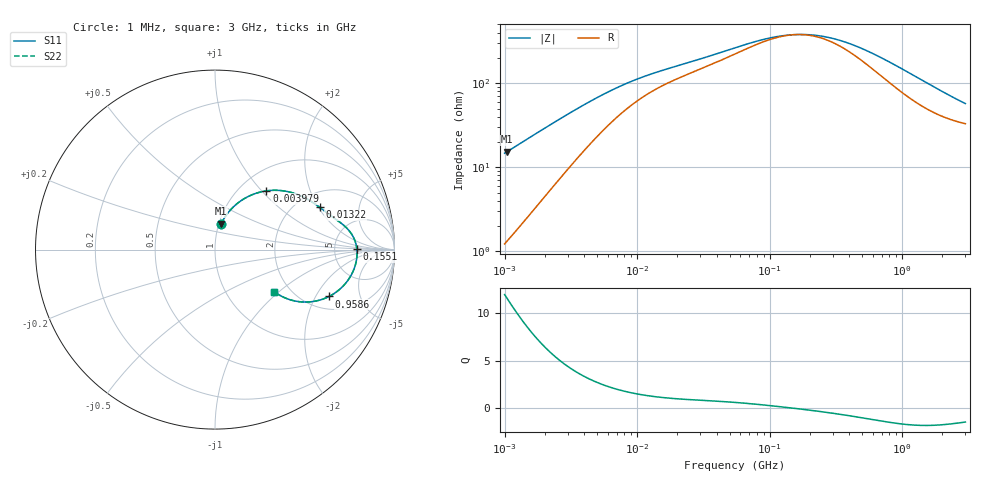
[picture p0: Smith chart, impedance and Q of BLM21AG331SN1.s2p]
! BLM21AG331SN1
# Hz S RI R 50
!Freq.(Hz) S11(Real) S11(Imag) S21(Real) S21(Imag) S12(Real) S12(Imag) S22(Real) S22(Imag)
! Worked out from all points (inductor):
!   401 points, 1 MHz to 3 GHz, reference 50 ohm
!   read as one part in series: L = 2.32 uH near 1.041 MHz
!   highest Q = 11.5 at 1.041 MHz (marker M1), where L = 2.33 uH
!   self-resonance near 157.2 MHz
!   S11 on the Smith chart (normalised r, x): 1 MHz: 1.02, +0.29; 3.979 MHz: 1.32, +1.06; 13.22 MHz: 2.63, +2.05; 155.1 MHz: 8.55, +0.07; 958.6 MHz: 2.63, -2.60; 3 GHz: 1.66, -0.93
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1000000  0.0324 0.1401  0.9676 -0.1401  0.9676 -0.1401  0.0324 0.1401
1040844  0.0349 0.1452  0.9651 -0.1452  0.9651 -0.1452  0.0349 0.1452
2014875  0.1114 0.2461  0.8886 -0.2461  0.8886 -0.2461  0.1114 0.2461
2720446  0.1769 0.2917  0.8231 -0.2917  0.8231 -0.2917  0.1769 0.2917
3823119  0.2742 0.3253  0.7258 -0.3253  0.7258 -0.3253  0.2742 0.3253
3979270  0.2866 0.3272  0.7134 -0.3272  0.7134 -0.3272  0.2866 0.3272
5372736  0.3806 0.3274  0.6194 -0.3274  0.6194 -0.3274  0.3806 0.3274
7550455  0.4751 0.3009  0.5249 -0.3009  0.5249 -0.3009  0.4751 0.3009
1.322427e7  0.5823 0.236  0.4177 -0.236  0.4177 -0.236  0.5823 0.236
1.461624e7  0.5963 0.2253  0.4037 -0.2253  0.4037 -0.2253  0.5963 0.2253
5.477226e7  0.7396 0.1139  0.2604 -0.1139  0.2604 -0.1139  0.7396 0.1139
9.984923e7  0.7789 0.0515  0.2211 -0.0515  0.2211 -0.0515  0.7789 0.0515
1.550909e8  0.7906 0.00155  0.2094 -0.00155  0.2094 -0.00155  0.7906 0.00155
2.094008e8  0.7911 -0.0344  0.2089 0.0344  0.2089 0.0344  0.7911 -0.0344
2.771263e8  0.7859 -0.0707  0.2141 0.0707  0.2141 0.0707  0.7859 -0.0707
3.667557e8  0.7736 -0.1106  0.2264 0.1106  0.2264 0.1106  0.7736 -0.1106
5.583748e8  0.7357 -0.1778  0.2643 0.1778  0.2643 0.1778  0.7357 -0.1778
8.005644e8  0.6761 -0.2362  0.3239 0.2362  0.3239 0.2362  0.6761 -0.2362
9.585869e8  0.6353 -0.2611  0.3647 0.2611  0.3647 0.2611  0.6353 -0.2611
1.268618e9  0.5592 -0.287  0.4408 0.287  0.4408 0.287  0.5592 -0.287
1.645649e9  0.482 -0.2914  0.518 0.2914  0.518 0.2914  0.482 -0.2914
3e9  0.3307 -0.2353  0.6693 0.2353  0.6693 0.2353  0.3307 -0.2353
